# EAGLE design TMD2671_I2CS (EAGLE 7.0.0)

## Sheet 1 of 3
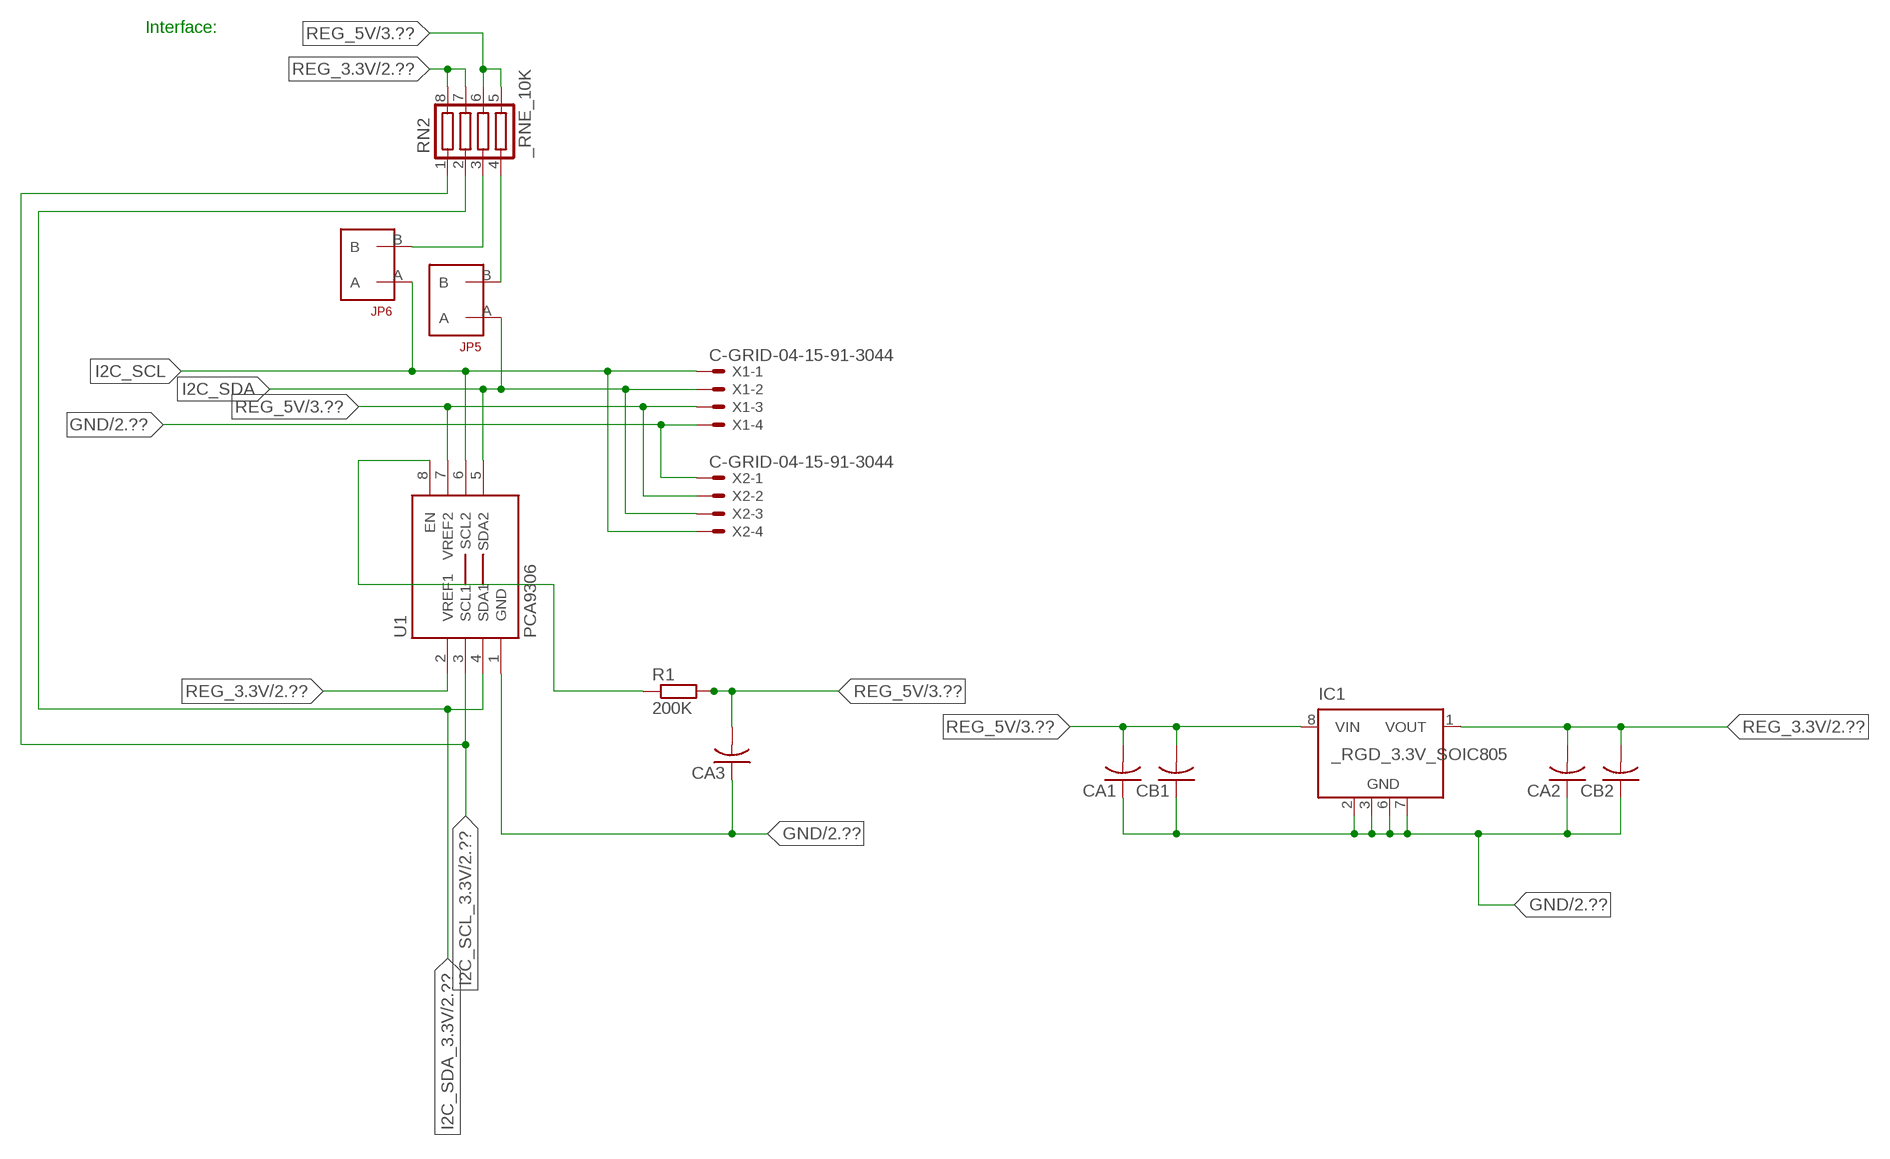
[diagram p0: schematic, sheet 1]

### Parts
CA1  CC1206KRX7R9BB104  [.1UF]
CA2  CC1206KRX7R9BB104  [.1UF]
CA3  CC1206KRX7R9BB104  [.1UF]
CB1  TMK316F106ZL-TC1206K  [TMK316F106ZL-T]
CB2  TMK316F106ZL-TC1206K  [TMK316F106ZL-T]
IC1  _RGD_3.3V_SOIC805  [_RGC_3.3V_SOIC8]
JP5  JUMPER_1X2_2MM  [JUMPER_1X2_2MM]
JP6  JUMPER_1X2_2MM  [JUMPER_1X2_2MM]
R1  200K  RESISTOR_SMT-0603  [R603]
RN2  _RNE_10K  [RNE]
U1  PCA9306  PCA9306_NCD  [PSOP-8]
X1  C-GRID-04-15-91-3044  [15-91-04]
X2  C-GRID-04-15-91-3044  [15-91-04]

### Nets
GND: CA1.1 CA2.1 CA3.1 CB1.1 CB2.1 IC1.2(GND) IC1.3(GND) IC1.6(GND) IC1.7(GND) U1.1(GND) X1.4 X2.1 ; also sheet 2,3
I2C_SCL: JP6.A U1.6(SCL2) X1.1 X2.4
I2C_SCL_3.3V: RN2.1 U1.3(SCL1) ; also sheet 2
I2C_SDA: JP5.A U1.5(SDA2) X1.2 X2.3
I2C_SDA_3.3V: RN2.2 U1.4(SDA1) ; also sheet 2
N$1: JP6.B RN2.3
N$2: JP5.B RN2.4
N$14: R1.1 U1.8(EN)
REG_3.3V: CA2.2 CB2.2 IC1.1(VOUT) RN2.7 RN2.8 U1.2(VREF1) ; also sheet 2
REG_5V: CA1.2 CA3.2 CB1.2 IC1.8(VIN) R1.2 RN2.5 RN2.6 U1.7(VREF2) X1.3 X2.2 ; also sheet 3
Unconnected: IC1.4(NC) IC1.5(NC)

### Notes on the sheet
- Interface:

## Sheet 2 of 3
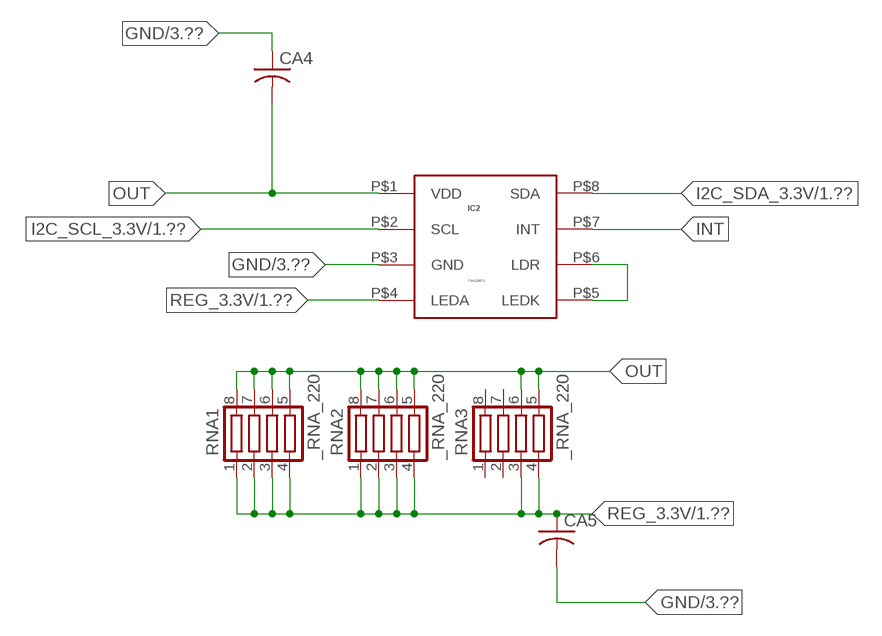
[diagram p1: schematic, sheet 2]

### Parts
CA4  _CA_.10UF_50VC1206K  [_CA_.1UF_50V]
CA5  _CA_.10UF_50VC1206K  [_CA_.1UF_50V]
IC2  TMD2671  TMD2771  [TMD2771]
RNA1  _RNA_220  [RNA]
RNA2  _RNA_220  [RNA]
RNA3  _RNA_220  [RNA]

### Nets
GND: CA4.1 CA5.2 IC2.P$3(GND) ; also sheet 1,3
I2C_SCL_3.3V: IC2.P$2(SCL) ; also sheet 1
I2C_SDA_3.3V: IC2.P$8(SDA) ; also sheet 1
INT: IC2.P$7(INT)
N$18: IC2.P$5(LEDK) IC2.P$6(LDR)
OUT: CA4.2 IC2.P$1(VDD) RNA1.5 RNA1.6 RNA1.7 RNA1.8 RNA2.5 RNA2.6 RNA2.7 RNA2.8 RNA3.5 RNA3.6
REG_3.3V: CA5.1 IC2.P$4(LEDA) RNA1.1 RNA1.2 RNA1.3 RNA1.4 RNA2.1 RNA2.2 RNA2.3 RNA2.4 RNA3.3 RNA3.4 ; also sheet 1
Unconnected: RNA3.1 RNA3.2 RNA3.7 RNA3.8

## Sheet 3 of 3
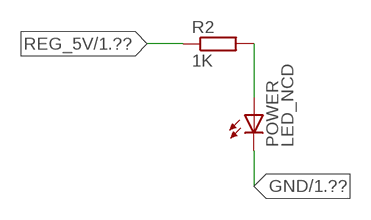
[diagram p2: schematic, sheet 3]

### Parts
POWER  LED_NCD  [CHIPLED_0603]
R2  1K  RESISTOR_SMT-0402  [R402]

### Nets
GND: POWER.C ; also sheet 1,2
N$4: POWER.A R2.2
REG_5V: R2.1 ; also sheet 1

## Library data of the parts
CA1-CA3 = NCD_ULTIMATE_LIBRARY:CC1206KRX7R9BB104: Capacitor CA .1uF 50V SMT C1206K CC1206KRX7R9BB104
CA4 CA5 = NCD_ULTIMATE_LIBRARY:_CA_.10UF_50V: Capacitor .1uF SMT
CB1 CB2 = NCD_ULTIMATE_LIBRARY:TMK316F106ZL-T: Capacitor CB 10uF SMT 1206 TMK316F106ZL-T
IC1 = NCD_ULTIMATE_LIBRARY:_RGD_3.3V_SOIC8: Regulator Linear 3.3V Chip Positive VOLTAGE REGULATOR Digikey 497-1199-2-ND/L78L33ACD13TR
IC2 = NCD_ULTIMATE_bhaskar:TMD2771: PROXIMITY DETECTOR DGTL Digikey TMD27711-TTR-ND/TMD27711
JP5 JP6 = NCD_ULTIMATE_CONNECTORS:JUMPER_1X2_2MM
POWER = NCD_ULTIMATE_LIBRARY:LED_NCD: LED Digikey 754-1132-2-ND/APT2012SRCPRV
R1 R2 = NCD_ULTIMATE_LIBRARY:RESISTOR_SMT: NCD Resistor
RN2 = NCD_ULTIMATE_LIBRARY:_RNE_10K: Resistor Array RNE SMT 10K x 4 Single Resistor Source: http://www.ctscorp.com/components/Datasheets/CTSChipArrayDs.pdf Digikey 742C083103JPTR-ND/742C083103JP; OC_FARNELL: unknown; OC_NEWARK: unknown
RNA1-RNA3 = NCD_ULTIMATE_LIBRARY:_RNA_220: Resistor Array RNA SMT 220 x 4 Single Resistor Source: http://www.ctscorp.com/components/Datasheets/CTSChipArrayDs.pdf Digikey 742C083221JPTR-ND/742C083221JP; OC_FARNELL: unknown; OC_NEWARK: unknown
U1 = NCD_ULTIMATE_LIBRARY:PCA9306_NCD: NCD Bidirectional I2C level shifter. NOT compatible with all available part number pinout schemes- DOUBLE CHECK!!!; PROD_ID: IC-10023
X1 X2 = NCD_ULTIMATE_CONNECTORS:C-GRID-04: CONNECTOR 4-Pos I2C wire to board 2.54 mm (0.100") pitch header Digikey WM1342-ND/0015912045; OC_FARNELL: unknown; OC_NEWARK: unknown

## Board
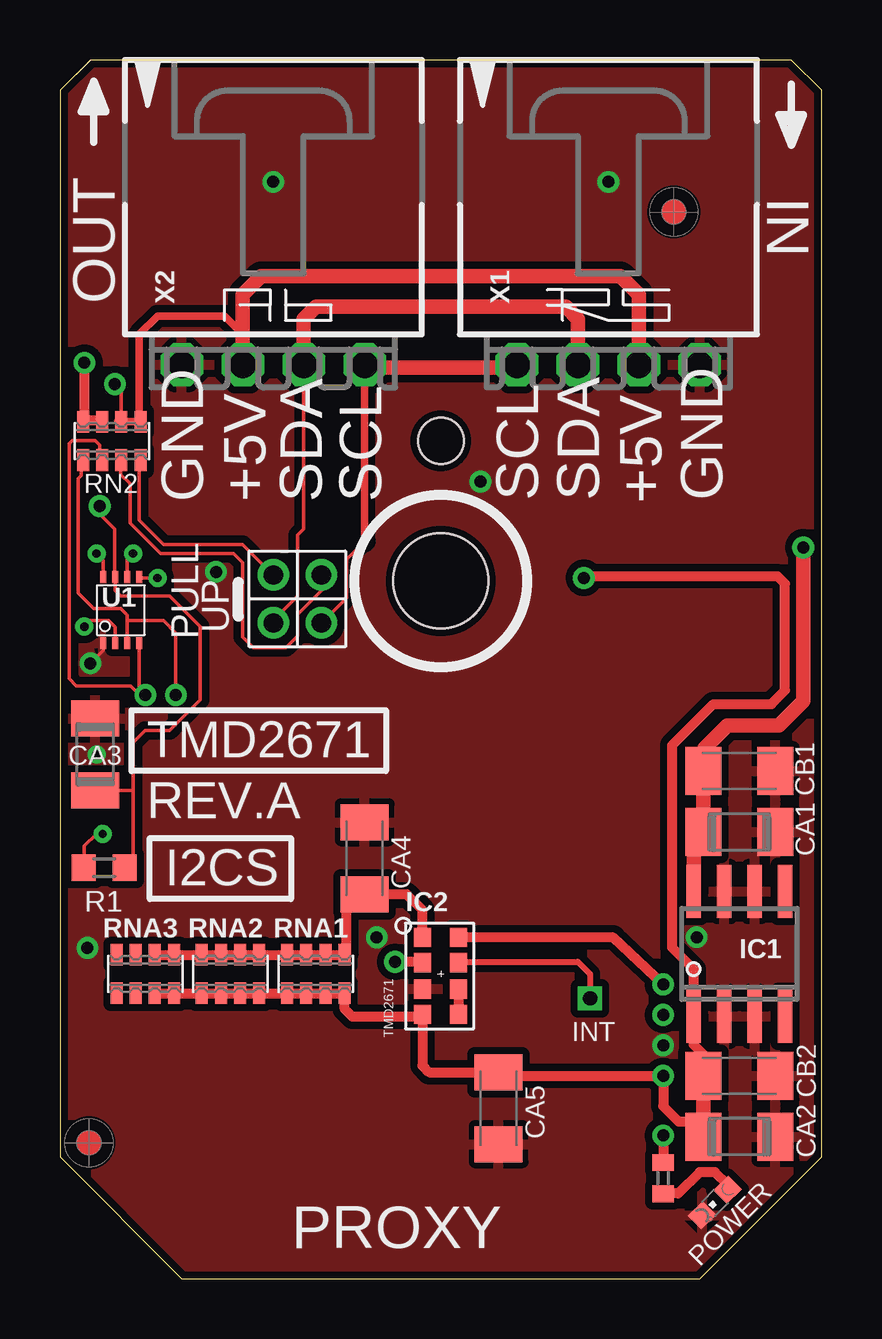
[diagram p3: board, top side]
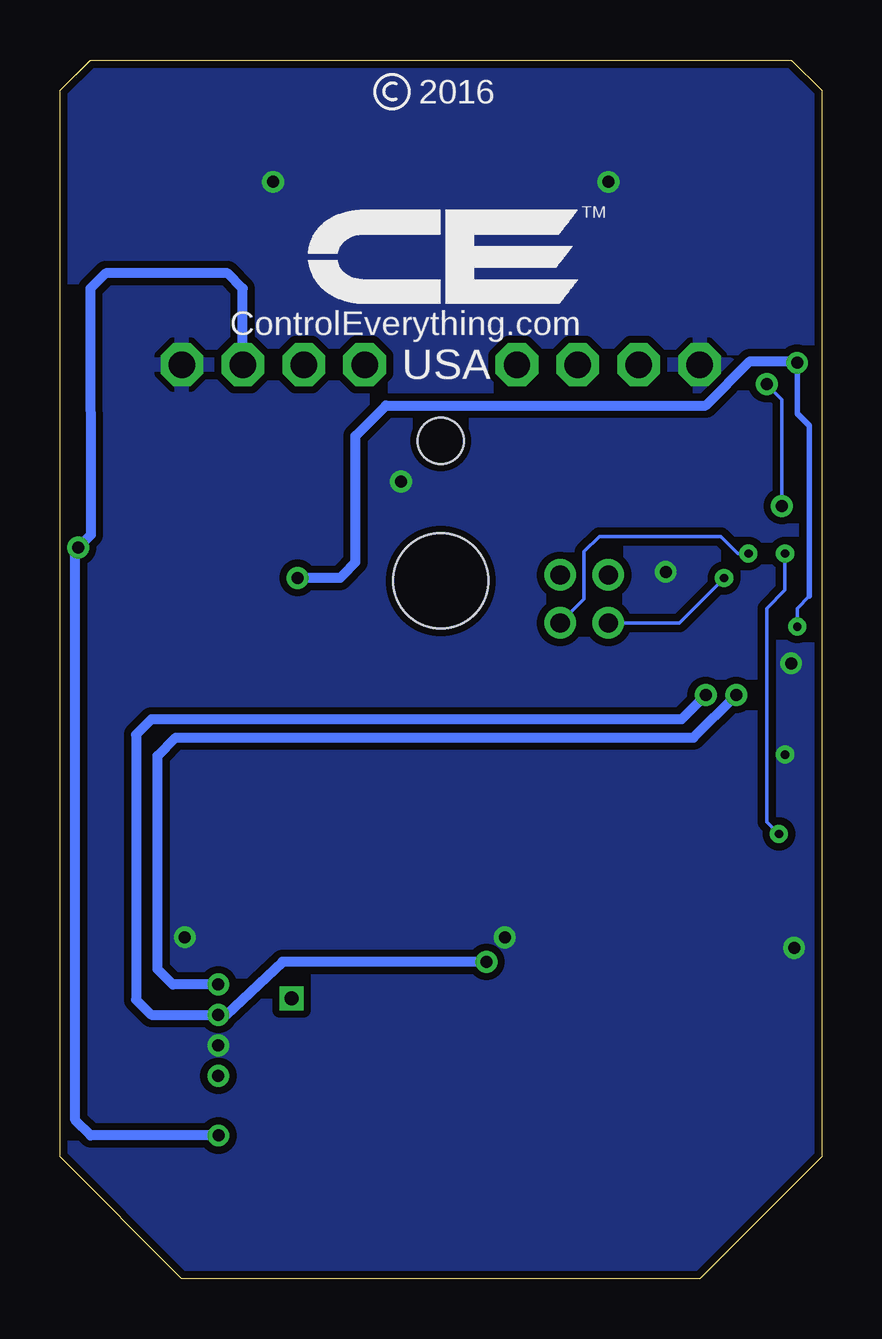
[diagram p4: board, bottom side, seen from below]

Size 31.75 x 50.8 mm. Coordinates in mm from the lower left corner, seen from the top.
Outline: 31.75,5.08 31.75,49.53 30.48,50.8 1.27,50.8 0,49.53 0,5.08 5.08,0 26.67,0 31.75,5.08
Outline: 31.75,5.08 31.75,49.53 30.48,50.8 1.27,50.8 0,49.53 0,5.08 5.08,0 26.67,0 31.75,5.08
Copper layers (1*16): Top 0.035mm / dielectric 1.5mm / Bottom 0.035mm
Design rules "default": minimum track width 5mil, minimum drill 24mil, track to track 5mil, track to pad 5mil, pad to pad 5mil, via to via 5mil, smd to smd 5mil, copper to edge 10mil, drill to drill 8mil, minimum pad ring 10mil, minimum via ring 8mil, stop-mask expansion 2mil, vias tented up to drill 0mil, thermal gap 10mil
Holes 3.96 mm at 15.88,29.08
Holes 1.91 mm at 15.88,34.93

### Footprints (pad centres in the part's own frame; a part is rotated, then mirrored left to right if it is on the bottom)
.1UF = smd 1.5 x 2: 1 -1.5,0; 2 1.5,0
_CA_.1UF_50V = smd 1.5 x 2: 1 -1.5,0; 2 1.5,0
TMK316F106ZL-T = smd 1.5 x 2: 1 -1.5,0; 2 1.5,0
_RGC_3.3V_SOIC8 = smd 0.6 x 2.2: 1 -1.905,-2.6; 2 -0.635,-2.6; 3 0.635,-2.6; 4 1.905,-2.6; 5 1.905,2.6; 6 0.635,2.6; 7 -0.635,2.6; 8 -1.905,2.6
TMD2771 = smd 0.7 x 0.8: P$1 -2.54,1.905; P$2 -2.54,0.855; P$3 -2.54,-0.245; P$4 -2.54,-1.295; P$5 -1.04,-1.295; P$6 -1.04,-0.245; P$7 -1.04,0.855; P$8 -1.04,1.905
JUMPER_1X2_2MM = drill 0.8: A 0,2; B 0,0
CHIPLED_0603 = smd 0.8 x 0.876: A 0,-0.75; C 0,0.75
R603 = smd 1 x 1.1: 1 -0.85,0; 2 0.85,0
R402 = smd 0.7 x 0.9: 1 -0.65,0; 2 0.65,0
RNE = smd 0.5 x 0.9: 1 -1.2,-0.8; 2 -0.4,-0.8; 3 0.4,-0.8; 4 1.2,-0.8; 5 1.2,0.8; 6 0.4,0.8; 7 -0.4,0.8; 8 -1.2,0.8
RNA = smd 0.5 x 0.9: 1 -1.2,-0.8; 2 -0.4,-0.8; 3 0.4,-0.8; 4 1.2,-0.8; 5 1.2,0.8; 6 0.4,0.8; 7 -0.4,0.8; 8 -1.2,0.8
PSOP-8 = smd 0.25 x 0.5: 1 -0.73,-1.37; 2 -0.23,-1.37; 3 0.27,-1.37; 4 0.77,-1.37; 5 0.77,1.38; 6 0.27,1.38; 7 -0.23,1.38; 8 -0.73,1.38
15-91-04 = drill 1.1 pad 1.778 octagon: 1 -3.81,-7.62; 2 -1.27,-7.62; 3 1.27,-7.62; 4 3.81,-7.62

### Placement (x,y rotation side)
CA1  28.32,18.62 180 top
CA2  28.32,5.92 180 top
CA3  1.46,21.86 270 top
CA4  12.7,17.53 270 top
CA5  18.29,7.11 270 top
CB1  28.32,21.16 180 top
CB2  28.32,8.46 180 top
IC1  28.32,13.54 0 top
IC2  17.65,12.32 0 top
JP5  8.89,29.34 180 top
JP6  10.9,29.34 180 top
POWER  27.3,3.18 135 top
R1  1.84,17.13 0 top
R2  25.15,4.19 270 top
RN2  2.16,34.93 0 top
RNA1  10.67,12.7 0 top
RNA2  7.11,12.7 0 top
RNA3  3.56,12.7 0 top
U1  2.54,27.86 0 top
U$5  [VISION_REF10]  1.21,5.66 90 top
U$28  [VISION_REF10]  25.59,44.46 90 top
X1  22.86,45.72 0 top
X2  8.89,45.72 0 top

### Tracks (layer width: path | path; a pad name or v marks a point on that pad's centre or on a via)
GND  (via drill 0.35, 0.5)
  Top 0.152: CA3.1 1.52,23.42 1.52,23.62 | v1.27,25.65 1.81,26.19 U1.1
  other vias: 8.89,45.72 22.86,45.72 25.15,9.73 17.53,33.22 26.55,14.24 1.15,13.79 6.5,29.46 13.21,14.22 1.52,21.84
  pour Top (isolate 0.305): -1.27,0 -1.27,50.8 33.02,50.8 33.02,0
  pour Bottom (isolate 0.305): -5.08,0 -5.08,50.8 35.56,50.8 35.56,0
I2C_SCL  (via drill 0.35)
  Top 0.152: 12.7,30.73 11.94,29.97 11.94,28.38 JP6.A | v3.05,30.23 2.81,29.99 U1.6
  Top 0.305: 12.7,30.73 X2.4
  Top 0.406: X2.4 12.7,37.97 | 19.05,37.97 X1.1
  Top 0.61: 12.7,37.97 19.05,37.97
  Bottom 0.152: JP6.A 9.91,28.33 9.91,30.3 9.27,30.94 4.19,30.94 3.48,30.23 v3.05,30.23
I2C_SCL_3.3V  (via drill 0.5)
  Top 0.152: RN2.1 0.89,34.07 0.89,33.48 0.77,33.35 0.77,28.59 1.41,27.94 2.54,27.94 2.81,27.67 2.81,27.43 | 2.81,27.43 U1.3 | v4.83,24.33 v4.83,24.34 4.83,26.92 4.32,27.43 2.81,27.43
  Top 0.406: IC2.P$2 15.08,13.21 v13.97,13.21
  Bottom 0.406: v4.83,24.33 5.84,23.32 27.94,23.32 28.58,22.68 28.58,11.63 27.94,11 v25.15,11 24.82,11 22.48,13.21 v13.97,13.21
I2C_SDA  (via drill 0.35)
  Top 0.152: JP5.A 8.89,27.44 9.91,28.45 9.91,30.99 10.16,31.24 10.16,34.92 X2.3 | U1.5 3.34,29.21 v4.06,29.21
  Top 0.61: X2.3 10.16,40.01 10.67,40.51 21.09,40.51 21.59,40.01 X1.2
  Bottom 0.152: v4.06,29.21 5.94,27.34 JP5.A
I2C_SDA_3.3V  (via drill 0.5)
  Top 0.152: RN2.2 1.65,34.14 1.65,34.75 1.46,34.94 0.51,34.94 0.38,34.81 0.38,26.37 0.38,26.36 0.38,25.02 0.69,24.71 2.95,24.71 3.33,24.33 v3.56,24.33 3.31,24.58 U1.4
  Top 0.406: v25.15,12.27 23.07,14.22 IC2.P$8
  Bottom 0.406: v25.15,12.27 27.05,12.27 27.69,12.9 27.69,21.79 26.93,22.56 5.34,22.56 v3.56,24.33
INT  (via drill 0.6)
  Top 0.254: IC2.P$7 16.9,13.21 21.59,13.21 22.1,12.7 v22.1,11.68
N$1
  Top 0.152: JP6.B 10.92,29.31 10.92,28.7 9.91,27.69 9.91,26.8 9.42,26.31 8.06,26.31 7.62,26.75 7.62,29.84 7.24,30.23 4.19,30.23 2.92,31.5 2.92,33.15 2.54,33.53 2.54,34.1 RN2.3
  Top 0.305: 2.54,34.02 RN2.3
N$2
  Top 0.152: JP5.B 7.62,30.61 4.32,30.61 3.3,31.62 3.3,34.07 RN2.4
  Top 0.305: 3.37,33.88 RN2.4
N$4
  Top 0.406: POWER.A 27.84,3.92 27.3,4.45 26.67,4.45 25.78,3.56 25.16,3.56 R2.2
N$14  (via drill 0.35)
  Top 0.152: R1.1 1.02,17.16 1.02,18.03 1.52,18.54 v1.78,18.54 | v1.52,30.23 1.81,29.94 U1.8
  Bottom 0.152: v1.78,18.54 2.29,19.05 2.29,27.94 1.52,28.7 v1.52,30.23
N$18
  Top 0.406: IC2.P$6 IC2.P$5
OUT
  Top 0.406: RNA3.6 RNA3.5 RNA2.8 RNA2.7 RNA2.6 RNA2.5 RNA1.8 RNA1.7 RNA1.6 RNA1.5 11.94,13.57 11.94,15.75 12.22,16.03 CA4.2 14.45,16.03 15.11,15.37 IC2.P$1
REG_3.3V  (via drill 0.35, 0.5)
  Top 0.152: v1.02,27.18 1.27,27.43 2.03,27.43 2.31,27.16 U1.2
  Top 0.406: CB2.2 26.82,9.35 26.42,9.75 26.42,10.36 | 26.82,6.55 25.78,6.55 25.15,7.19 v25.15,8.46 18.7,8.46 CA5.1 15.39,8.61 15.11,8.89 IC2.P$4 15.21,10.92 12.19,10.92 11.87,11.25 RNA1.4 RNA1.3 RNA1.2 RNA1.1 RNA2.4 RNA2.3 RNA2.2 RNA2.1 RNA3.4 RNA3.3 | IC1.1 26.42,12.9 25.53,13.79 25.53,22.24 27.24,23.95 29.66,23.95 30.23,24.52 30.23,28.97 29.91,29.29 21.92,29.29 v21.84,29.21 | 26.52,5.62 CA2.2 | v1.02,38.18 1.02,35.78 | 1.02,35.78 RN2.8 | 1.02,35.78 1.7,35.78 RN2.7
  Top 0.61: CB2.2 26.82,6.55 CA2.2 | 26.42,10.36 IC1.1
  Bottom 0.152: 0.51,28.45 1.02,27.94 v1.02,27.18
  Bottom 0.229: 0.51,28.45 0.51,35.56 1.02,36.07 v1.02,38.18
  Bottom 0.406: v1.02,38.18 1.08,38.24 2.99,38.24 4.83,36.4 18.16,36.4 19.43,35.13 19.43,29.87 19.94,29.34 20.07,29.21 v21.84,29.21
REG_5V  (via drill 0.5)
  Top 0.152: RN2.6 2.56,37.01 v2.29,37.29 | R1.2 3.05,17.49 3.05,20.36 | 3.05,20.36 3.05,22.35 3.56,22.86 4.57,22.86 5.84,24.13 5.84,27.18 4.57,28.45 2.54,28.45 2.31,28.68 U1.7 2.29,29.27 2.29,31.24 1.65,31.87 v1.65,32.21 | CA3.2 3.05,20.36
  Top 0.305: 7.62,39.37 7.5,39.37 | 2.42,35.74 RN2.6 RN2.5 3.3,35.8 3.3,39.37 4.07,40.13 6.86,40.13 7.62,39.37 | X2.2 7.62,39.37
  Top 0.406: v25.15,5.97 R2.1
  Top 0.61: X1.3 24.13,41.02 23.37,41.78 8.38,41.78 7.62,41.02 X2.2 | IC1.8 26.42,18.21 CA1.2 CB1.2 26.86,21.2 26.86,22.11 27.82,23.06 29.98,23.06 30.99,24.08 v30.99,30.48
  Bottom 0.152: v1.65,32.21 1.65,36.65 v2.29,37.29
  Bottom 0.406: X1.3 24.13,41.28 24.77,41.91 29.84,41.91 30.48,41.27 30.47,31 v30.99,30.48 31.12,30.36 31.12,6.6 30.48,5.97 v25.15,5.97

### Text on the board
tNames: IN | OUT | GND | +5V | SDA | SCL | SCL | SDA | +5V | GND | UP | PULL | TMD2671 | REV.A | I2CS | INT | PROXY
bNames: 2016 | TM | ControlEverything.com | USA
